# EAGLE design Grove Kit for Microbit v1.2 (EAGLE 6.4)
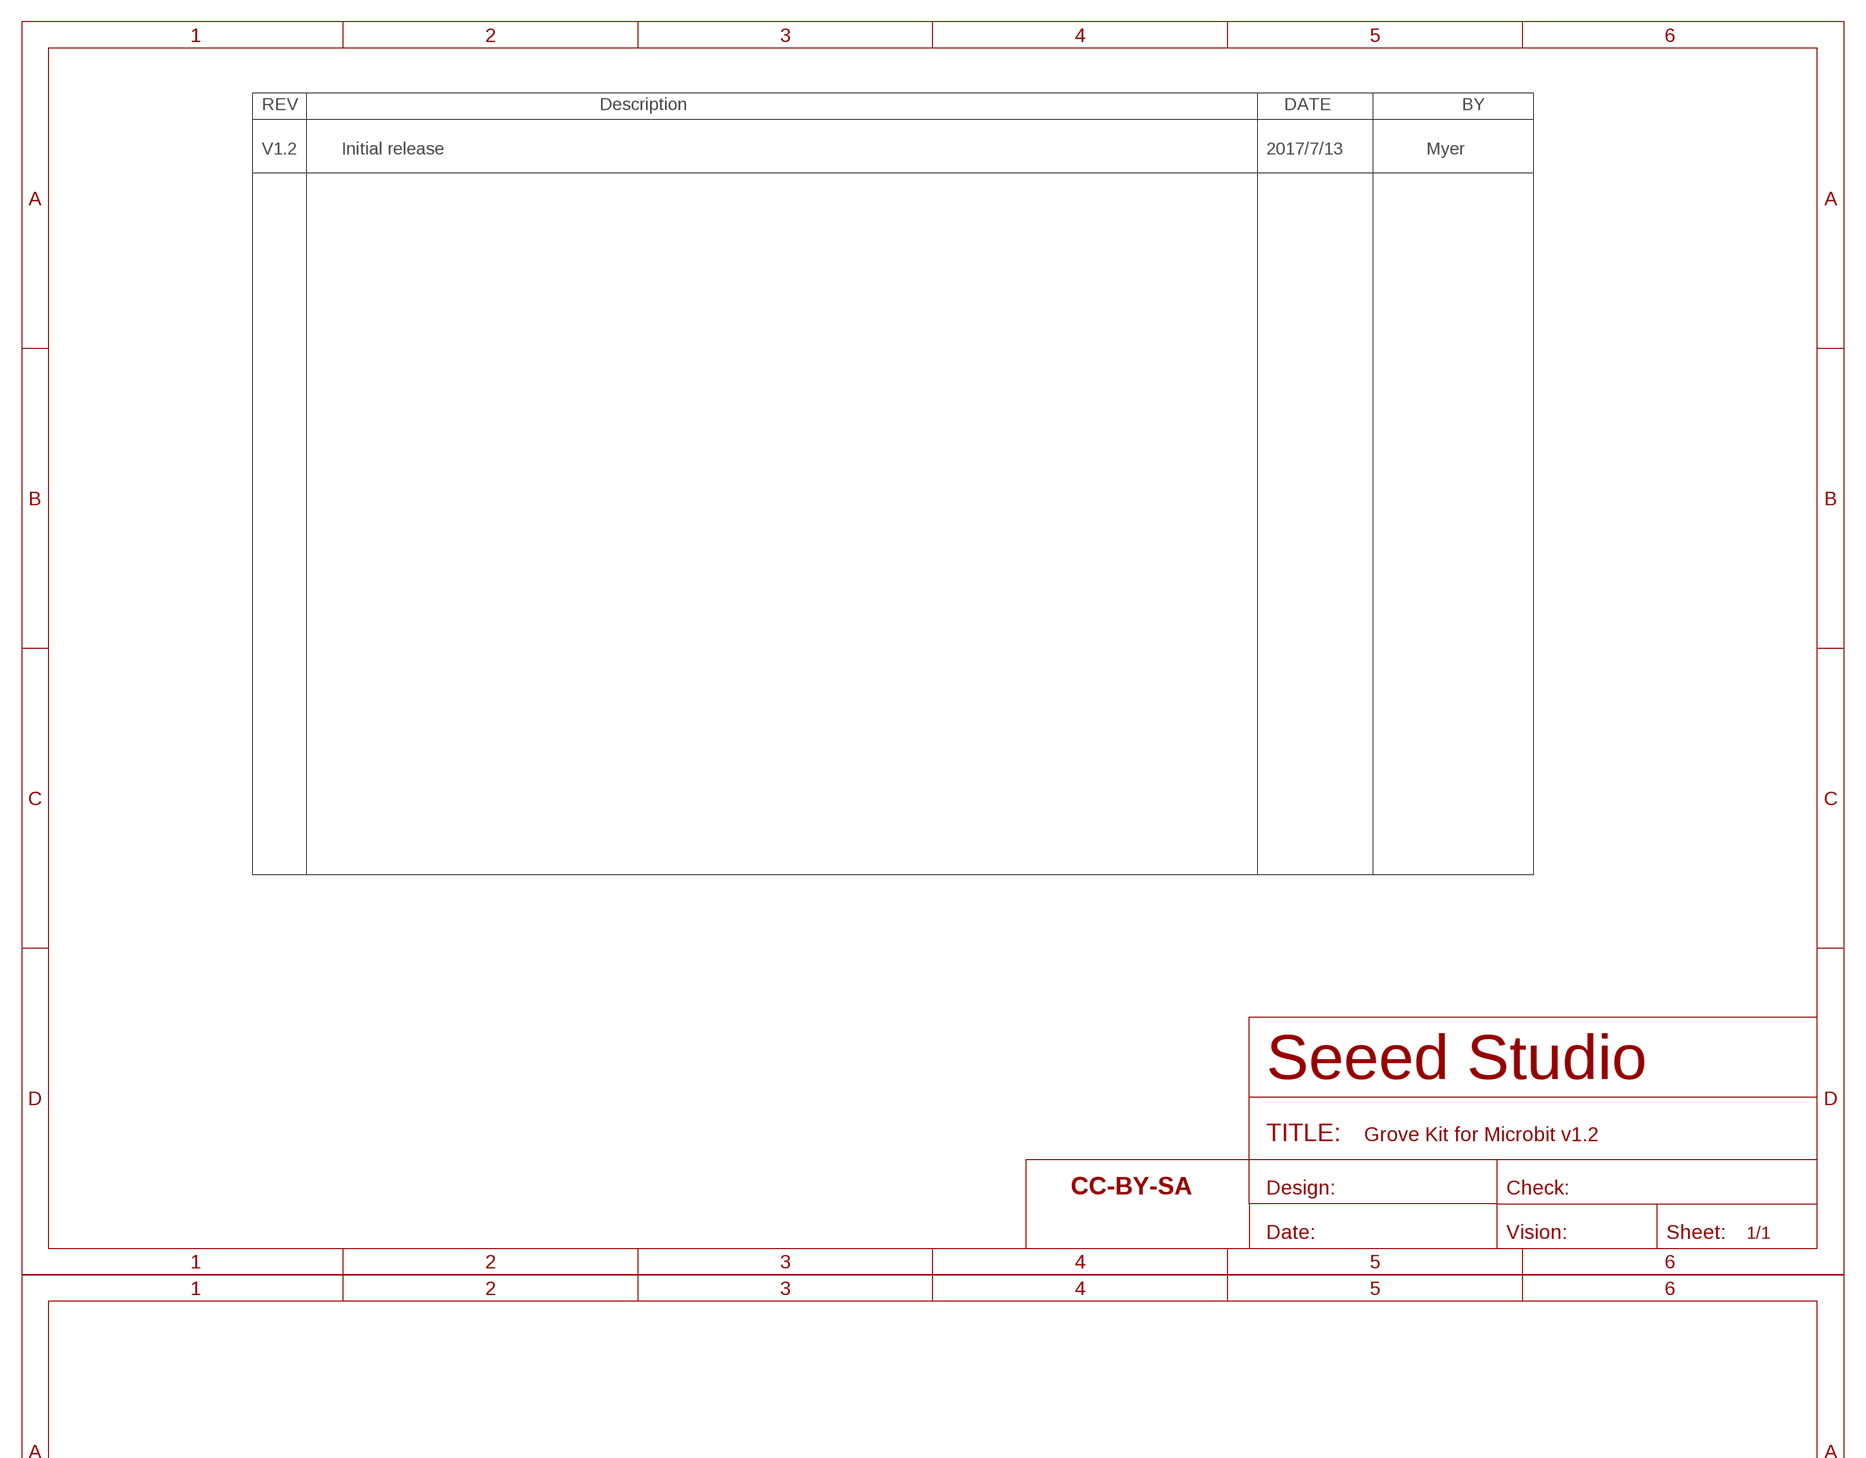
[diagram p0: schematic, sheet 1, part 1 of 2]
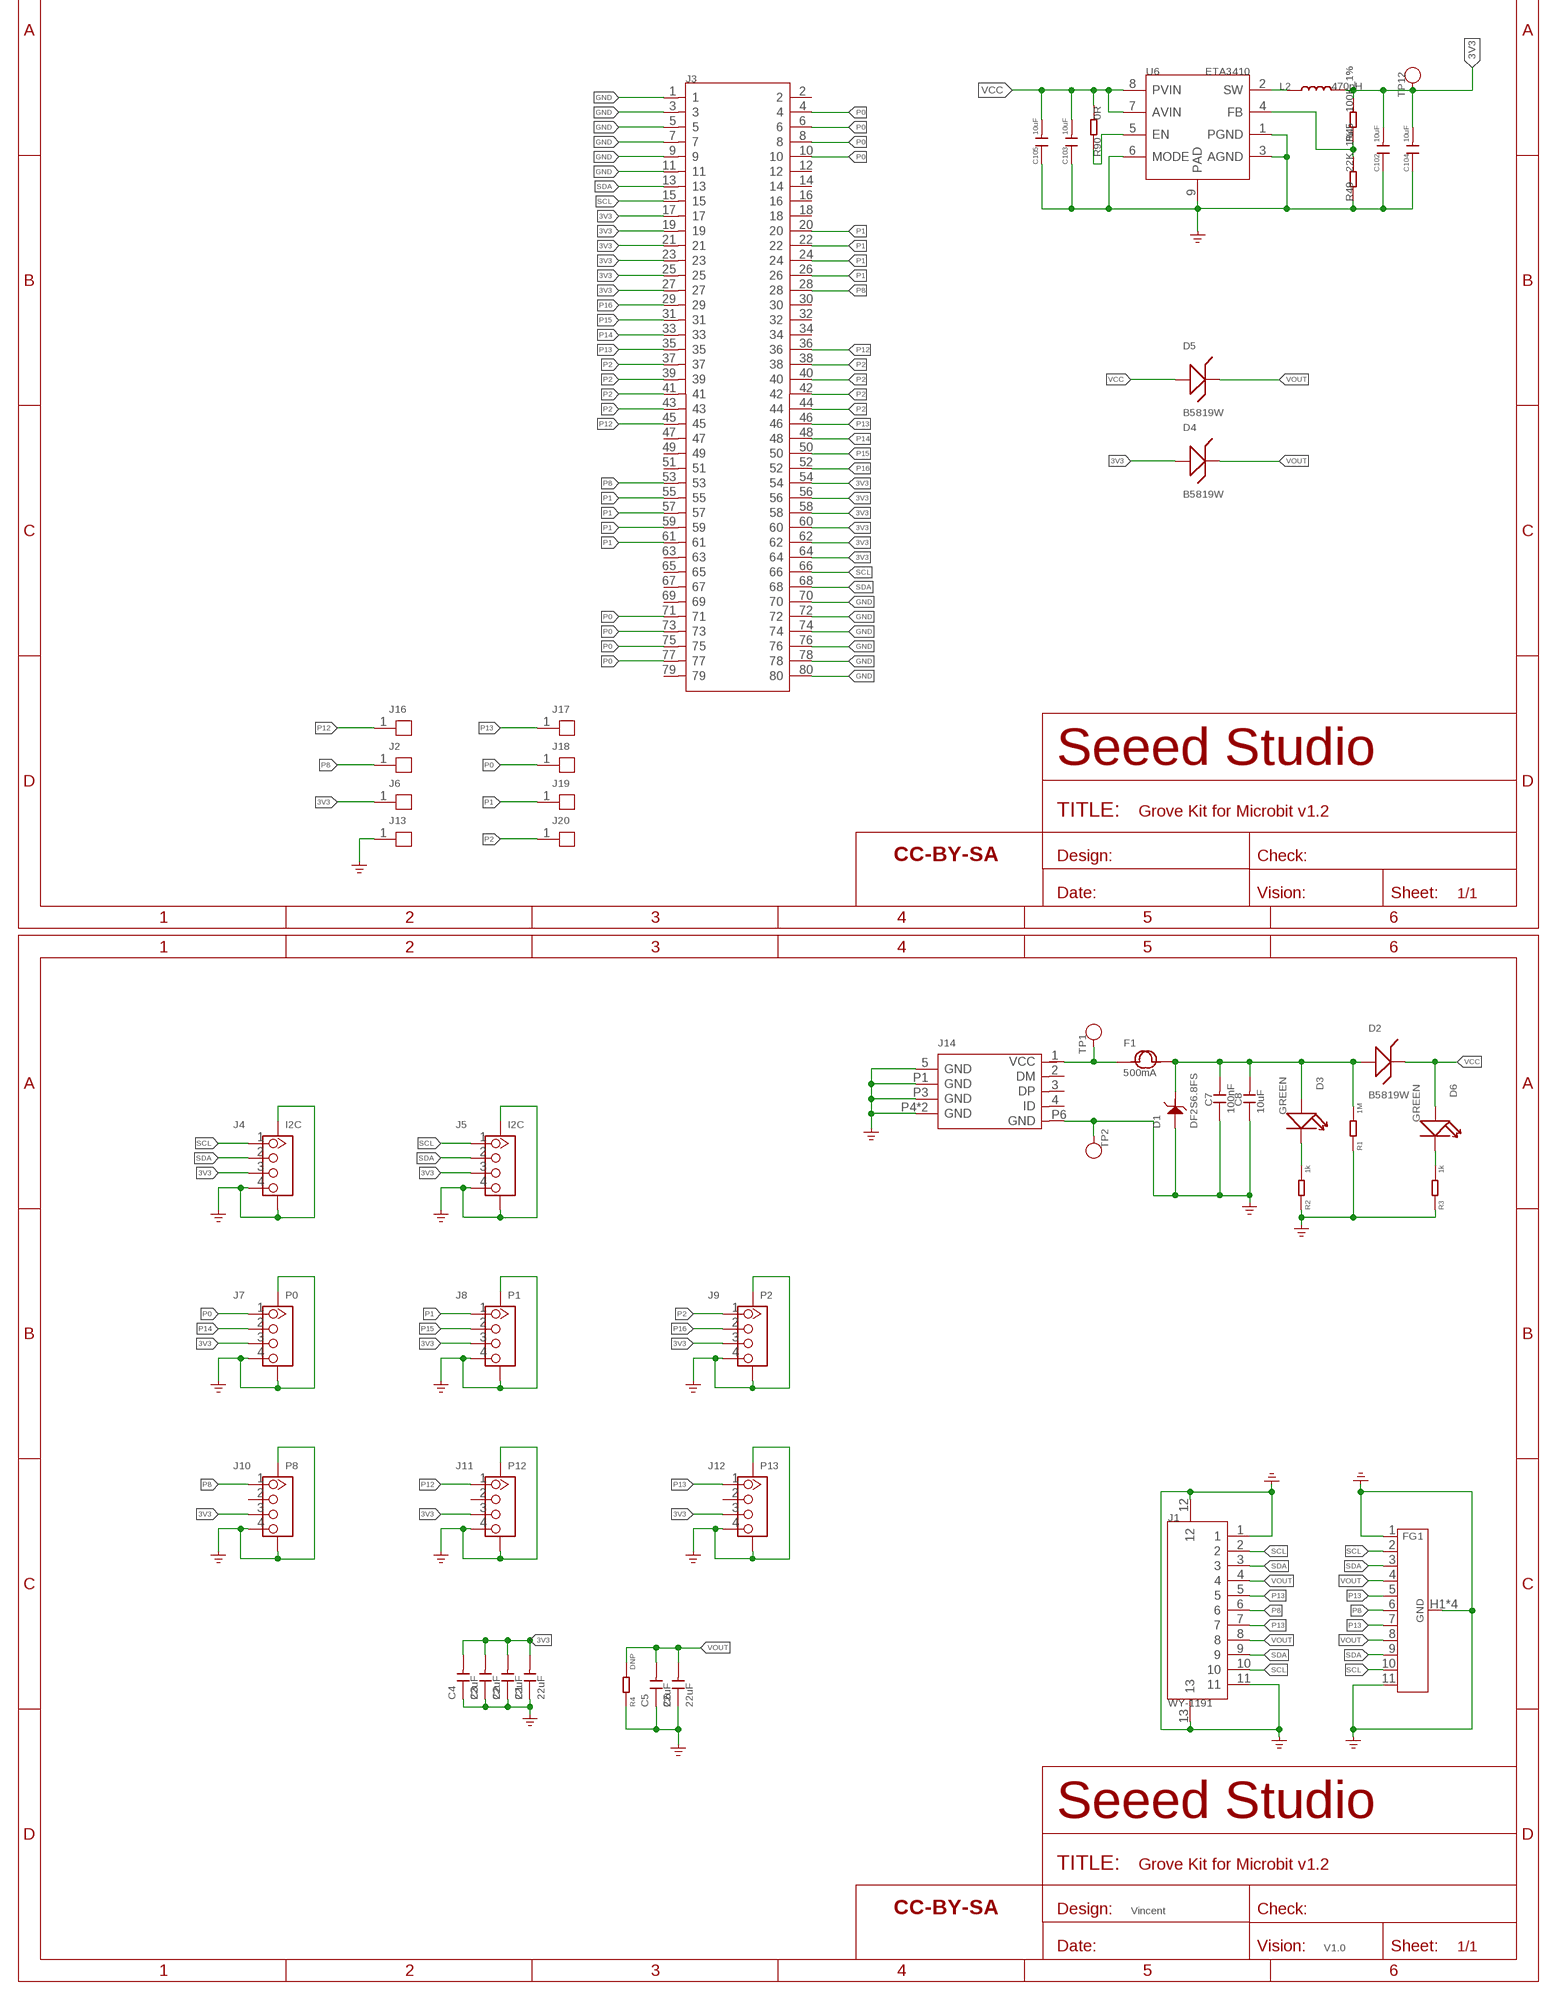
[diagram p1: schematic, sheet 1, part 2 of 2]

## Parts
C1  22uF  CAP-0805  [C0805]
C2  22uF  CAP-0805  [C0805]
C3  22uF  CAP-0805  [C0805]
C4  22uF  CAP-0805  [C0805]
C5  22uF  CAP-0805  [C0805]
C6  22uF  CAP-0805  [C0805]
C7  100nF  C-0402  [C0402]
C8  10uF  C-0603  [C0603]
C102  10uF  C-0603  [C0603]
C103  10uF  C-0603  [C0603]
C104  10uF  C-0603  [C0603]
C105  10uF  C-0603  [C0603]
D1  DF2S6.8FS  D-ESD-2P'DF2S6.8FS'  [SOD-923]
D2  B5819W  D-ZENER-2P'MMSZ4689-V'  [SOD-123]
D3  GREEN  LED-0402  [LED-0402]
D4  B5819W  D-ZENER-2P'MMSZ4689-V'  [SOD-123]
D5  B5819W  D-ZENER-2P'MMSZ4689-V'  [SOD-123]
D6  GREEN  LED-0402  [LED-0402]
F1  500mA  FUSE'1206'  [F1206]
FG1  HALF_FINGER  [HALF_FINGER]
FR1  SEEEDSTUDIO-OPEN-SCH-FRAME  [SEEEDSTUDIO-PCB-FRAME]
FR2  SEEEDSTUDIO-OPEN-SCH-FRAME  [SEEEDSTUDIO-PCB-FRAME]
FR3  SEEEDSTUDIO-OPEN-SCH-FRAME  [SEEEDSTUDIO-PCB-FRAME]
J1  WY-1191  HEADER-11P-SMD  [H11P-SMD-1.0-13.5X4.35X3.1MM]
J2  HEADER-1P-3.9MM  [1P-DIP-8X5MM]
J3  CONNECTOR-MICRO-BIT-2X40P  [CONNECTOR2X40P-1.27-57X14]
J4  I2C  GROVE-CONNECTOR-SMD'90D'  [HW4-SMD-2.0-90D]
J5  I2C  GROVE-CONNECTOR-SMD'90D'  [HW4-SMD-2.0-90D]
J6  HEADER-1P-3.9MM  [1P-DIP-8X5MM]
J7  P0  GROVE-CONNECTOR-SMD'90D'  [HW4-SMD-2.0-90D]
J8  P1  GROVE-CONNECTOR-SMD'90D'  [HW4-SMD-2.0-90D]
J9  P2  GROVE-CONNECTOR-SMD'90D'  [HW4-SMD-2.0-90D]
J10  P8  GROVE-CONNECTOR-SMD'90D'  [HW4-SMD-2.0-90D]
J11  P12  GROVE-CONNECTOR-SMD'90D'  [HW4-SMD-2.0-90D]
J12  P13  GROVE-CONNECTOR-SMD'90D'  [HW4-SMD-2.0-90D]
J13  HEADER-1P-3.9MM  [1P-DIP-8X5MM]
J14  MICRO-USB5+4P  [MICRO-USB5+5P-SMD-0.65-7.2X5.06MM]
J16  HEADER-1P-3.9MM  [1P-DIP-8X5MM]
J17  HEADER-1P-3.9MM  [1P-DIP-8X5MM]
J18  HEADER-1P-3.9MM  [1P-DIP-8X5MM]
J19  HEADER-1P-3.9MM  [1P-DIP-8X5MM]
J20  HEADER-1P-3.9MM  [1P-DIP-8X5MM]
L2  470nH  L-MPM201610SR33_T  [L201610]
R1  1M  R-0402  [R0402]
R2  1k  R-0402  [R0402]
R3  1k  R-0402  [R0402]
R4  DNP  R-0402  [R0402]
R45  100K_1%  R-0402  [R0402]
R49  22K_1%  R-0402  [R0402]
R90  0R  R-0402  [R0402]
TP1  TEST-POINT'4545'  [TP-D45MIL]
TP2  TEST-POINT'4545'  [TP-D45MIL]
TP12  TEST-POINT'4545'  [TP-D45MIL]
U6  ETA3410  CONVERTER-ETA3410  [DFN8G-0.5-2X2MM]

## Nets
3V3: C1.2 C2.2 C3.2 C4.2 C102.2 C104.2 D4.+ J3.17 J3.19 J3.21 J3.23 J3.25 J3.27 J3.54 J3.56 J3.58 J3.60 J3.62 J3.64 J4.3 J5.3 J6.1 J7.3 J8.3 J9.3 J10.3 J11.3 J12.3 L2.2 R45.2 TP12.T
GND: C1.1 C2.1 C3.1 C4.1 C5.1 C6.1 C7.1 C8.1 C102.1 C103.1 C104.1 C105.1 D1.2 FG1.1 FG1.11 FG1.H1 FG1.H2 FG1.P2 FG1.P4 J1.1 J1.11 J1.12 J1.13 J3.1 J3.3 J3.5 J3.7 J3.9 J3.11 J3.70 J3.72 J3.74 J3.76 J3.78 J3.80 J4.4 J4.SS1 J4.SS2 J5.4 J5.SS1 J5.SS2 J7.4 J7.SS1 J7.SS2 J8.4 J8.SS1 J8.SS2 J9.4 J9.SS1 J9.SS2 J10.4 J10.SS1 J10.SS2 J11.4 J11.SS1 J11.SS2 J12.4 J12.SS1 J12.SS2 J13.1 J14.5(GND) J14.P1(GND) J14.P3(GND) J14.P4(GND) J14.P5(GND) J14.P6(GND) R1.1 R2.1 R3.1 R4.1 R49.1 TP2.T U6.1(PGND) U6.3(AGND) U6.6(MODE) U6.9(PAD) ; supply symbol labelled GND_POWER
N$1: D6.- R3.2
N$2: D3.- R2.2
N$3: C7.2 C8.2 D1.1 D2.+ D3.+ F1.2 R1.2
N$17: R90.1 U6.5(EN)
N$24: F1.1 J14.1(VCC) TP1.T
N$48: L2.1 U6.2(SW)
N$49: R45.1 R49.2 U6.4(FB)
P0: J3.4 J3.6 J3.8 J3.10 J3.71 J3.73 J3.75 J3.77 J7.1 J18.1
P1: J3.20 J3.22 J3.24 J3.26 J3.55 J3.57 J3.59 J3.61 J8.1 J19.1
P2: J3.37 J3.38 J3.39 J3.40 J3.41 J3.42 J3.43 J3.44 J9.1 J20.1
P8: FG1.6 J1.6 J2.1 J3.28 J3.53 J10.1
P12: J3.36 J3.45 J11.1 J16.1
P13: FG1.5 FG1.7 J1.5 J1.7 J3.35 J3.46 J12.1 J17.1
P14: J3.33 J3.48 J7.2
P15: J3.31 J3.50 J8.2
P16: J3.29 J3.52 J9.2
SCL: FG1.2 FG1.10 J1.2 J1.10 J3.15 J3.66 J4.1 J5.1
SDA: FG1.3 FG1.9 J1.3 J1.9 J3.13 J3.68 J4.2 J5.2
VCC: C103.2 C105.2 D2.- D5.+ D6.+ R90.2 U6.7(AVIN) U6.8(PVIN)
VOUT: C5.2 C6.2 D4.- D5.- FG1.4 FG1.8 J1.4 J1.8 R4.2
Unconnected: J3.2 J3.12 J3.14 J3.16 J3.18 J3.30 J3.32 J3.34 J3.47 J3.49 J3.51 J3.63 J3.65 J3.67 J3.69 J3.79 J10.2 J11.2 J12.2 J14.2(DM) J14.3(DP) J14.4(ID)

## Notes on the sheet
- V1.2 | Initial release | 2017/7/13 | Myer
- Vincent
- V1.0

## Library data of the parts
C1-C6 = Discrete-new:CAP: Ceramic Capacitors
C7 C8 C102-C105 = Discrete-small:C*: Ceramic Capacitors
D1 = Discrete-new:D-ESD-2P: SOD-923:304060009;SOD-123:304060001
D2 D4 D5 = Discrete-new:D-ZENER-2P: SOD-123:304030008;SOT-23:304030000
D3 D6 = Discrete-new:LED
F1 = Discrete-new:FUSE
FG1 = G2-Xadow3:HALF_FINGER
FR1-FR3 = moudle-new:SEEEDSTUDIO-OPEN-SCH-FRAME
J1 = Connector-new:HEADER-11P-SMD
J2 J6 J13 J16-J20 = Connector-new:HEADER-1P
J3 = Connector-new:CONNECTOR-MICRO-BIT-2X40P
J4 J5 J7-J12 = Connector-new:GROVE-CONNECTOR-SMD: 4P-SMD-2.0:320110030;4P-SMD-2.0-90D:320110032
J14 = Connector-new:MICRO-USB5+4P: 5+4P-SMD-0.65-B:320010000;5+2P-SMD-0.65-AB:340032001;5+5P-SMD-0.65-7.2X5.06MM:320010050;
L2 = Discrete-new:L
R1-R4 R45 R49 R90 = Discrete-small:R*
TP1 TP2 TP12 = Discrete-new:TEST-POINT; PARTNO: DNP
U6 = IC-new:CONVERTER-ETA3410: 3MHZ 2A High Step-Down Converter in DFN2x2-8L Package

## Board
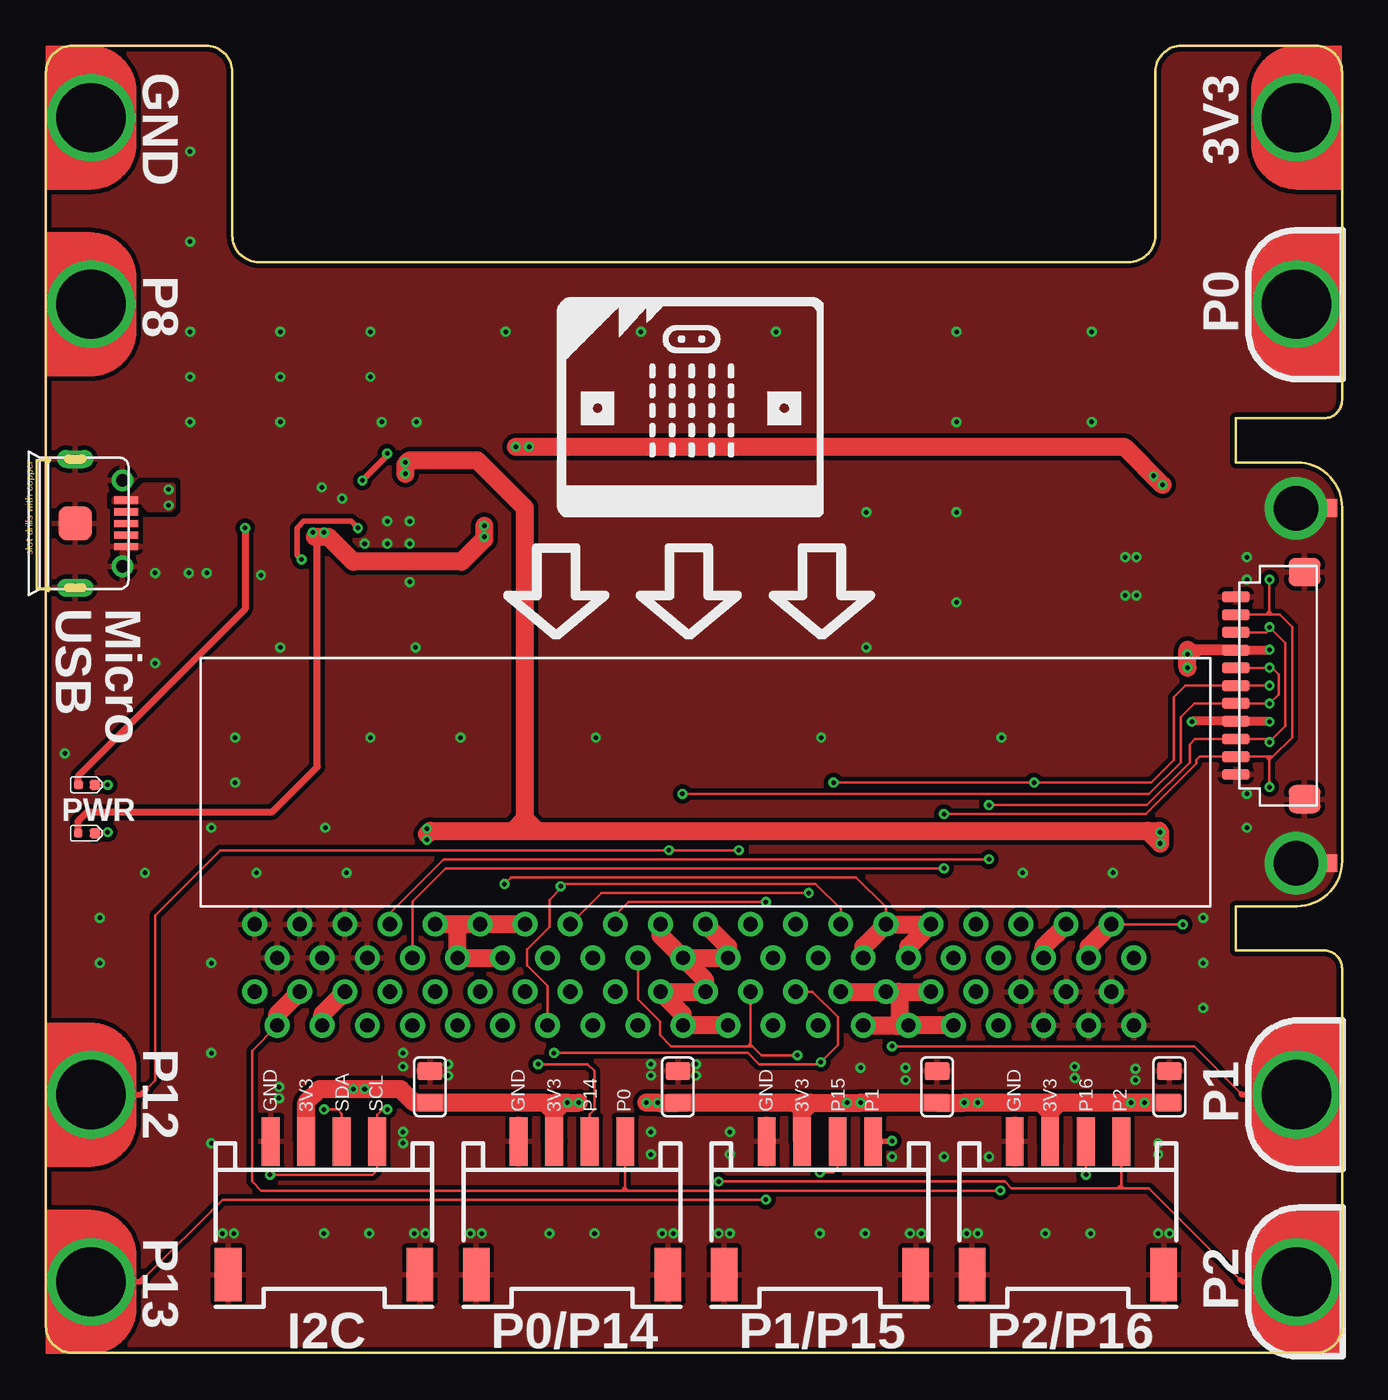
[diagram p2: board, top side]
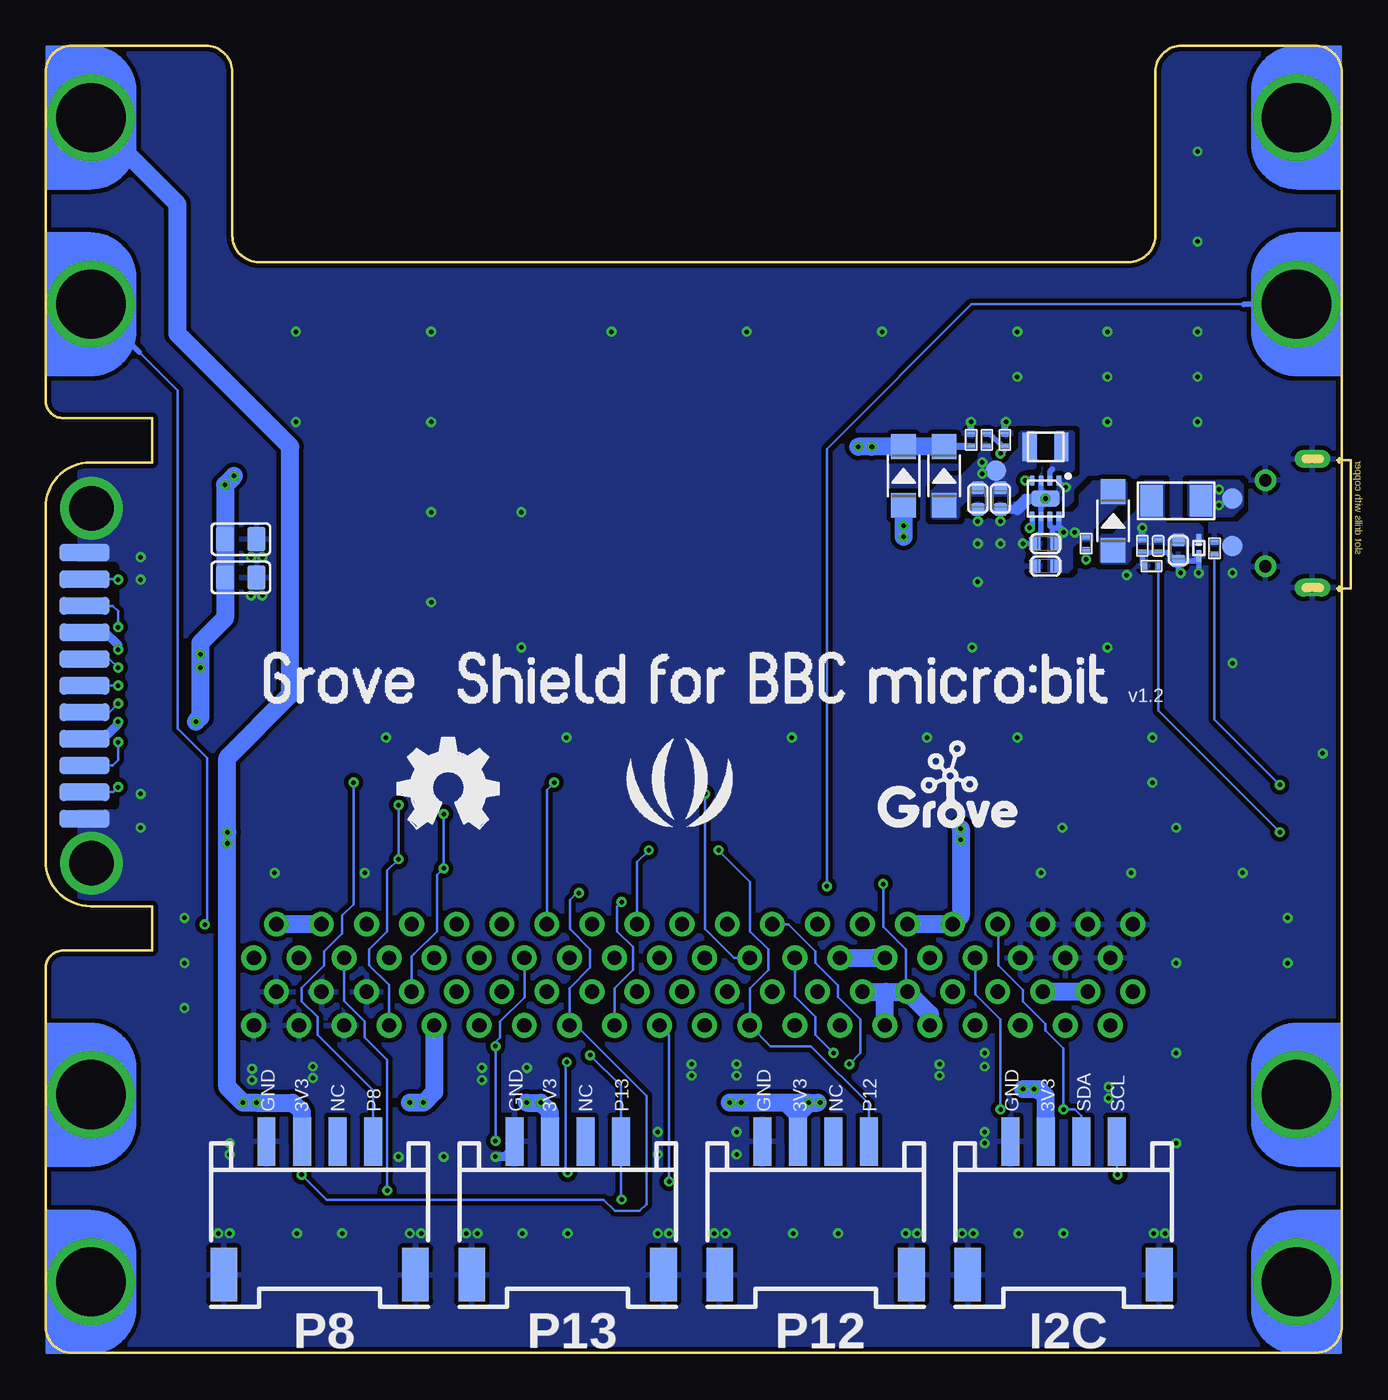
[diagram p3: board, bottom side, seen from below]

Size 73.03 x 73.65 mm. Coordinates in mm from the lower left corner, seen from the top.
Outline: 71.53,0 arc90 73.03,1.49 73.03,21.67 arc90 72.03,22.67 67.03,22.67 67.03,25.17 70.49,25.17 arc90 73.03,27.71 73.03,47.63 arc90 70.49,50.17 67.03,50.17 67.03,52.67 72.03,52.67 arc90 73.03,53.67 73.03,72.16 arc90 71.53,73.65 64,73.65 arc90 62.5,72.15 62.5,62.95 arc-90 61,61.45 12,61.45 arc-90 10.5,62.95 10.5,72.15 arc90 9,73.65 1.5,73.65 arc90 0,72.15
Outline: 0,72.14 0,1.5 arc90 1.5,0 71.54,0
Copper layers (1*16): Top 0.035mm / dielectric 1.5mm / Bottom 0.035mm
Design rules "SeeedStudio_2layer_DRU_no_angle_20140221 *": minimum track width 1mil, minimum drill 10mil, track to track 5mil, track to pad 5mil, pad to pad 5mil, via to via 5mil, smd to smd 0mil, copper to edge 10mil, drill to drill 10mil, minimum pad ring 10mil, minimum via ring 6mil, stop-mask expansion 2mil, vias tented up to drill 25mil, thermal gap 10mil
bRestrict: area 16.4,50.5 to 16.9,51.9

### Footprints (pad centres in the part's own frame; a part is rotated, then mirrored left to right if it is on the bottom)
C0805 = smd 1.397 x 1.016: 1 0,0.889; 2 0,-0.889
C0402 = smd 0.508 x 0.385: 1 0,0.383; 2 0,-0.383
C0603 = smd 0.762 x 0.696: 1 0,0.602; 2 0,-0.602
SOD-923 = smd 0.7 x 0.3: 1 -0.45,0; 2 0.45,0
SOD-123 = smd 1.397 x 1.397: + -1.651,0; - 1.651,0
LED-0402 = smd 0.5 x 0.5: + -0.463,0 | smd 0.58 x 0.58: - 0.468,0
F1206 = smd 1.27 x 1.778: 1 -1.397,0; 2 1.397,0
HALF_FINGER = smd 2.8 x 1 bottom: 1 3.8,7.5; 2 3.8,6; 3 3.8,4.5; 4 3.8,3; 5 3.8,1.5; 6 3.8,0; 7 3.8,-1.5; 8 3.8,-3; 9 3.8,-4.5; 10 3.8,-6; 11 3.8,-7.5 | drill 2.5 pad 3.516: H1 3.4,10; H2 3.4,-10 | smd 1.27 x 1: P2 5.1,10; P4 5.1,-10
H11P-SMD-1.0-13.5X4.35X3.1MM = smd 0.6 x 1.55: 1 -5,0; 2 -4,0; 3 -3,0; 4 -2,0; 5 -1,0; 6 0,0; 7 1,0; 8 2,0; 9 3,0; 10 4,0; 11 5,0 | smd 1.6 x 1.8: 12 -6.4,3.875; 13 6.4,3.875
1P-DIP-8X5MM = drill 3.9: 1 0,0
CONNECTOR2X40P-1.27-57X14 = drill 0.8 pad 1.4: 1 24.13,0; 2 24.13,3.8; 3 22.86,1.9; 4 22.86,5.7; 5 21.59,0; 6 21.59,3.8; 7 20.32,1.9; 8 20.32,5.7; 9 19.05,0; 10 19.05,3.8; 11 17.78,1.9; 12 17.78,5.7; 13 16.51,0; 14 16.51,3.8; 15 15.24,1.9; 16 15.24,5.7; 17 13.97,0; 18 13.97,3.8; 19 12.7,1.9; 20 12.7,5.7; 21 11.43,0; 22 11.43,3.8; 23 10.16,1.9; 24 10.16,5.7; 25 8.89,0; 26 8.89,3.8; 27 7.62,1.9; 28 7.62,5.7; 29 6.35,0; 30 6.35,3.8; 31 5.08,1.9; 32 5.08,5.7; 33 3.81,0; 34 3.81,3.8; 35 2.54,1.9; 36 2.54,5.7; 37 1.27,0; 38 1.27,3.8; 39 0,1.9; 40 0,5.7; 41 -1.27,0; 42 -1.27,3.8; 43 -2.54,1.9; 44 -2.54,5.7; 45 -3.81,0; 46 -3.81,3.8; 47 -5.08,1.9; 48 -5.08,5.7; 49 -6.35,0; 50 -6.35,3.8; 51 -7.62,1.9; 52 -7.62,5.7; 53 -8.89,0; 54 -8.89,3.8; 55 -10.16,1.9; 56 -10.16,5.7; 57 -11.43,0; 58 -11.43,3.8; 59 -12.7,1.9; 60 -12.7,5.7; 61 -13.97,0; 62 -13.97,3.8; 63 -15.24,1.9; 64 -15.24,5.7; 65 -16.51,0; 66 -16.51,3.8; 67 -17.78,1.9; 68 -17.78,5.7; 69 -19.05,0; 70 -19.05,3.8; 71 -20.32,1.9; 72 -20.32,5.7; 73 -21.59,0; 74 -21.59,3.8; 75 -22.86,1.9; 76 -22.86,5.7; 77 -24.13,0; 78 -24.13,3.8; 79 -25.4,1.9; 80 -25.4,5.7
HW4-SMD-2.0-90D = smd 1.01 x 2.74: 1 -3,-0.1; 2 -1,-0.1; 3 1,-0.1; 4 3,-0.1 | smd 1.5 x 3: SS1 -5.4,7.4; SS2 5.4,7.4
MICRO-USB5+5P-SMD-0.65-7.2X5.06MM = smd 0.4 x 1.35: 1 -1.3,2.875; 2 -0.65,2.875; 3 0,2.875; 4 0.65,2.875; 5 1.3,2.875 | smd 1.9 x 1.9: P1 0,0 | drill 0.508 pad 1.016 long: P3 -3.625,0; P4 3.625,0 | drill 0.7: P5 -2.425,2.65; P6 2.425,2.65
L201610 = smd 0.8 x 1.6: 1 -0.9,0; 2 0.9,0
R0402 = smd 0.508 x 0.385: 1 0,0.383; 2 0,-0.383
TP-D45MIL = smd 1.143 x 1.143: T 0,0
DFN8G-0.5-2X2MM = smd 0.6 x 0.3: 1 -1,0.75; 2 -1,0.25; 3 -1,-0.25; 4 -1,-0.75; 5 1,-0.75; 6 1,-0.25; 7 1,0.25; 8 1,0.75 | smd 0.9 x 1.6: 9 0,0

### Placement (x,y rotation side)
C1  35.61,14.99 0 top
C2  50.21,14.99 0 top
C3  21.64,14.99 0 top
C4  63.3,14.99 0 top
C5  62.03,43.69 270 bottom
C6  62.03,45.85 270 bottom
C7  10.34,45.47 180 bottom
C8  9.19,45.21 180 bottom
C102  20.5,48.13 180 bottom
C103  16.69,44.32 90 bottom
C104  19.23,48.13 180 bottom
C105  16.69,45.59 90 bottom
D1  8.05,45.34 270 bottom
D2  12.88,46.87 90 bottom
D3  2.29,32 0 top
D4  22.4,49.4 90 bottom
D5  24.69,49.4 90 bottom
D6  2.28,29.27 0 top
F1  9.32,48.01 180 bottom
FG1  67.03,37.59 0 top
FR1  not placed on the board
FR2  not placed on the board
FR3  not placed on the board
J1  67.03,37.59 270 top
J2  2.54,59.08 180 top
J3  37.16,18.45 0 top
J4  15.67,11.81 180 top
J5  15.67,11.81 180 bottom
J6  70.46,69.6 0 top
J7  29.64,11.81 180 top
J8  43.61,11.81 180 top
J9  57.58,11.81 180 top
J10  57.58,11.81 180 bottom
J11  29.64,11.81 180 bottom
J12  43.61,11.81 180 bottom
J13  2.54,69.6 180 top
J14  1.65,46.74 270 top
J16  2.54,14.55 180 top
J17  2.54,4 180 top
J18  70.46,59.08 0 top
J19  70.46,14.55 0 top
J20  70.46,4 0 top
L2  16.69,51.05 180 bottom
R1  11.24,45.47 180 bottom
R2  7.16,45.34 0 bottom
R3  10.72,44.33 90 bottom
R4  20.88,51.44 0 bottom
R45  19.99,51.44 0 bottom
R49  18.97,51.44 0 bottom
R90  14.4,45.59 180 bottom
TP1  6.16,48.13 180 bottom
TP2  6.16,45.47 180 bottom
TP12  19.48,49.72 180 bottom
U6  16.69,48.13 270 bottom
U$13  [OSHW_FILLX200_NOTEXT_TNAME]  53.18,29.56 0 bottom
U$14  [SEEED-SILK-TNAME-280*268MIL]  37.3,31.34 0 bottom

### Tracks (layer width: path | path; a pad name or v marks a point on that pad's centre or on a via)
3V3  (via drill 0.25 pad 0.51)
  Top 0.305: v21.46,28.9 21.46,29.21 | v21.46,29.54 21.46,29.26 21.49,29.24
  Top 1.016: 26.97,29.41 21.66,29.41 21.49,29.24 21.46,29.21 | 26.97,29.41 62.08,29.41 | 62.08,29.41 62.71,29.41 v62.79,29.34 v62.79,28.7 62.08,29.41 | J3.58 J3.62 23.19,24.12 23.16,24.15 | J3.56 J3.60 23.16,24.15 | J3.17 48.22,18.45 48.16,18.52 | 48.16,18.52 48.13,18.54 48.13,20.28 48.05,20.35 | 48.05,20.35 J3.23 J3.27 | 48.05,20.35 J3.19 | J3.25 47.93,18.45 | 48.02,18.45 J3.21 47.93,18.45 | 48.16,18.52 48.05,18.41 47.96,18.41 47.93,18.45 | 42.21,14.1 42.59,14.1 | 42.59,14.1 43.1,14.1 | J8.3 42.61,14.08 42.59,14.1 | 42.21,14.1 42.59,13.72 | 43.1,14.1 42.59,13.59 | v33.83,14.1 v34.47,14.1 C1.2 42.21,14.1 | 28.12,14.1 28.75,14.1 | 28.75,14.1 v29.39,14.1 | v29.39,14.1 v30.02,14.1 | J7.3 28.64,13.99 28.75,14.1 | 28.12,14.1 28.62,13.59 29.13,14.1 v29.39,14.1 | J4.3 14.67,14.11 15.42,14.86 v17.32,14.86 19.99,14.86 20.75,14.1 C3.2 28.12,14.1 | v61.14,14.1 56.69,14.1 | 56.69,14.1 56.06,14.1 | 56.06,14.1 v52.5,14.1 v51.74,14.1 C2.2 v45.9,14.1 43.1,14.1 | J9.3 56.58,13.99 56.69,14.1 | 56.06,14.1 56.44,13.72 | v61.14,14.1 57.07,14.1 56.69,13.72 | C4.2 v61.14,14.1 | 26.97,30.1 26.97,47.62 24.31,50.29 20.5,50.29 20.24,50.04 v20.24,49.53 | 26.97,30.1 26.97,29.41 | 26.97,30.1 26.34,29.46 | 26.97,30.1 27.61,29.46 | 23.16,24.15 J3.64 21.89,24.13
  Bottom 0.508: 29.51,14.1 v29.39,14.1
  Bottom 1.016: v52.5,14.1 v51.74,14.1 51.13,14.71 J3.17 | J3.60 J3.64 21.46,24.61 v21.46,29.54 | J3.54 26.34,22.25 | 26.34,22.25 J3.58 | J12.3 44.61,13.57 v45.13,14.1 v45.9,14.1 | J11.3 30.64,13.48 v30.02,14.1 | v30.02,14.1 29.51,14.1 | v30.02,14.1 31.29,14.1 | 31.29,14.1 v34.47,14.1 | 31.29,14.1 30.66,13.46 | J10.3 58.58,13.57 59.1,14.1 v61.14,14.1 v61.9,14.1 62.79,14.99 v62.79,29.34 62.79,33.53 59.23,37.08 59.23,51.05 65.58,57.4 65.58,64.71 J6.1 | J5.3 16.67,14.46 17.07,14.86 v17.32,14.86 v17.96,14.86 | 26.35,22.26 26.34,22.25
  other vias: 20.24,50.17
  pour Bottom (isolate 0.254, no thermals): 23.04,46.99 21.64,46.99 21.51,47.12 21.51,47.62 20.88,48.26 18.46,48.26 18.21,48.51 18.21,49.33 17.75,49.78 17.32,49.78 17.19,49.91 17.19,51.82 17.32,51.94 18.08,51.94 18.21,51.82 18.21,50.98 18.89,50.29 19.3,50.29 19.41,50.29 19.61,50.48 19.61,51.13 19.79,51.31 20.21,51.31 20.5,51.02 20.5,50.37 21.46,49.4 22.27,49.4 23.16,48.51 23.16,47.12
GND  (via drill 0.25 pad 0.51)
  Bottom 0.305: 17.29,45.88 17.32,45.85 | 17.29,45.88 C105.1 v17.96,45.59 | 17.29,45.88 16.94,46.23 U6.6 16.94,47.88 U6.9 16.94,48.38 U6.3 | U6.1 15.94,49.03 15.67,48.77 v15.54,48.77 | R3.1 11.24,44.47 R1.1 C7.1 9.83,45.08 9.35,44.61 C8.1 | D1.2 8.05,44.83 | 8.05,44.83 v8.05,43.94 | C8.1 8.27,44.61 8.05,44.83 | C8.1 9.19,44.07 v9.07,43.94
  Bottom 0.406: R4.1 v20.88,52.45 | R49.1 18.97,52.39 v18.91,52.45
  Bottom 0.508: C104.1 18.43,47.53 17.83,48.13 17.57,48.13 | 17.57,48.13 U6.9 | 17.57,48.13 18.27,47.43 | J12.4 46.61,11.61 47.17,11.05 v47.67,11.05
  other vias: 19.23,46.86 20.5,46.86 19.23,45.59 20.5,45.59 20.5,43.43 16.69,48.13 20.11,16.89 20.11,16.13 22.65,15.62 22.65,16.26 61.39,16 61.39,15.37 34.09,15.62 34.09,16.26 36.62,16.26 36.62,15.62 57.96,15.49 57.96,16.13 48.44,15.37 48.44,16.07 38.53,12.45 38.53,11.18 50.6,11.05 53.14,11.05 20.11,12.45 20.11,11.81 13.13,14.99 13.13,14.35 9.96,6.73 10.59,6.73 20.75,6.73 21.38,6.73 23.93,6.73 24.56,6.73 34.09,12.45 34.09,11.18 34.72,6.73 35.36,6.73 37.9,6.73 38.53,6.73 48.69,6.73 49.33,6.73 51.87,6.73 52.5,6.73 62.66,6.73 63.3,6.73 62.66,11.81 62.66,11.18 67.67,31.5 67.67,29.59 67.67,43.56 67.67,44.83 45.9,16.07 9.32,16.89 9.32,11.81 9.32,29.59 8.12,62.61 8.12,67.69 55.04,27.05 60.12,27.05 65.2,24.51 65.2,21.97 65.2,19.43 9.32,21.97 61.45,42.67 60.81,42.67 60.81,44.83 61.45,44.83 6.15,43.94 12.11,43.82 8.12,57.53 13.2,57.53 18.28,57.53 18.28,54.99 13.2,54.99 8.12,54.99 8.12,52.45 13.2,52.45 25.9,57.53 33.52,57.53 41.14,57.53 51.3,57.53 58.92,57.53 58.92,52.45 51.3,52.45 51.3,47.37 51.3,42.29 15.74,29.59 18.28,34.67 23.36,34.67 30.98,34.67 43.68,34.67 53.84,34.67 3.04,24.51 5.58,27.05 3.04,21.97 10.66,32.13 10.66,34.67 13.2,39.75 20.82,39.75 46.22,47.37 46.22,39.75 6.15,38.86 1.06,33.78 15.67,6.73 28.37,6.73 30.91,6.73 43.61,6.73 46.15,6.73 56.31,6.73 58.85,6.73 18.21,6.73 11.86,27.05 16.94,27.05
  pour Top (isolate 0.254, rank 6): -0.21,74.04 73.45,74.04 73.45,-0.25 -0.21,-0.25
  pour Bottom (isolate 0.254, rank 6): -0.21,74.04 73.45,74.04 73.45,-0.25 -0.21,-0.25
N$1  (via drill 0.25 pad 0.51)
  Top 0.127: D6.- 3.41,29.27 v3.48,29.34
  Bottom 0.127: R3.2 10.33,36.19 v3.48,29.34
N$2  (via drill 0.25 pad 0.51)
  Top 0.127: v3.48,32 D3.-
  Bottom 0.127: R2.2 7.16,35.69 v3.48,32
N$3  (via drill 0.25 pad 0.51)
  Top 0.406: v11.22,46.48 11.22,41.91 1.95,32.64 1.83,32.51 1.82,32.51 D3.+
  Bottom 0.406: R1.2 v11.24,46.47 v11.22,46.48
  pour Bottom (isolate 0.254, no thermals): 10.08,49.15 11.1,49.15 11.48,48.77 11.48,47.55 12.93,46.1 13.51,46.1 13.64,45.97 13.64,44.58 13.51,44.45 12.11,44.45 11.86,44.7 11.86,45.34 11.73,45.47 7.92,45.47 7.8,45.59 7.8,46.48 8.05,46.74 9.83,46.74 9.96,46.86 9.96,49.02
N$17  (via drill 0.25 pad 0.51)
  Top 0.305: v14.4,44.7 14.15,44.96 14.15,46.48 14.53,46.86 17.19,46.86 v17.57,46.48
  Bottom 0.305: R90.1 v14.4,44.7 | U6.5 17.44,46.62 v17.57,46.48
N$24  (via drill 0.25 pad 0.51)
  other vias: 6.91,48.64 6.91,47.75
  pour Bottom (isolate 0.254, no thermals): 8.3,47.12 6.15,47.12 5.51,47.75 5.51,48.9 5.76,49.15 8.56,49.15 8.69,49.02 8.69,47.24 8.56,47.12
  pour Top (isolate 0.254, no thermals): 3.86,48.26 4.75,48.26 5.51,49.02 7.16,49.02 7.29,48.9 7.29,47.62 7.03,47.37 5.76,47.37 5.38,47.75 3.86,47.75 3.73,47.88 3.73,48.13
N$48
  Bottom 0.305: U6.2 16.44,49.65 16.3,49.78
  pour Bottom (isolate 0.254, no thermals): 16.3,49.66 15.16,49.66 15.04,49.78 15.04,51.82 15.16,51.94 16.05,51.94 16.18,51.82 16.18,50.29 16.43,50.04 16.43,49.78
N$49  (via drill 0.25 pad 0.51)
  Top 0.305: v17.83,49.15 19.23,50.55 v19.23,50.67
  Bottom 0.305: U6.4 17.81,49.13 v17.83,49.15 | R45.1 19.86,51.82 19.1,51.05 R49.2 18.97,50.93 v19.23,50.67
P0  (via drill 0.25 pad 0.51)
  Top 0.127: v53.77,9.14 32.81,9.14 | 32.81,9.14 32.69,9.14 | 32.69,9.14 32.43,9.14 | 32.43,9.14 12.11,9.14 11.61,9.65 11.61,17.03 J3.77 | J7.1 32.64,9.35 | 32.64,9.32 32.64,9.19 32.69,9.14 | 32.64,9.35 32.43,9.14 | 32.64,9.35 32.64,9.32 | 32.64,9.32 32.81,9.14 | J3.4 64.04,24.15 v64.06,24.13
  Top 1.016: J3.77 13.03,19.08 J3.75 | J3.73 15.57,19.08 J3.71 | J3.10 56.21,22.88 J3.8 | J3.6 58.75,22.88 J3.4
  Bottom 0.127: v53.77,9.14 53.77,16.51 55.04,17.78 55.04,18.67 56.21,19.84 J3.10 | v64.06,24.13 63.93,24.26 63.93,33.53 65.58,35.18 65.58,54.23 67.74,56.39 | J18.1 70.44,59.06 70.41,59.06 68.63,57.28
  Bottom 0.305: 68.63,57.28 67.74,56.39
  Bottom 1.016: J3.75 J3.71 | J3.8 J3.4
P1  (via drill 0.25 pad 0.51)
  Top 0.127: v25.83,26.42 26.21,26.8 45.64,26.8 47.32,25.12 J3.24 | v47.67,17.27 64.69,17.27 67.36,14.61 | J19.1 68.85,14.55
  Top 0.305: J8.1 47.65,11.91 v47.67,11.94 | 68.85,14.55 67.42,14.55 67.36,14.61
  Top 1.016: J3.26 46.05,22.88 J3.24 J3.20 48.59,22.88 J3.22
  Bottom 0.127: v25.83,26.42 25.83,24 24.56,22.73 24.56,20.45 24.49,20.39 J3.59 | J3.26 46.05,20.04 47.42,18.67 47.42,17.78 47.67,17.53 v47.67,17.27 v47.67,11.94
  Bottom 1.016: J3.61 23.19,19.08 J3.59 | J3.55 25.7,20.35 | 25.7,20.35 24.53,20.35 24.49,20.39 | J3.57 25.73,20.32 25.7,20.35
P2  (via drill 0.25 pad 0.51)
  Top 0.127: J9.1 60.58,9.48 | 60.58,9.45 60.58,9.32 60.63,9.27 | v37.9,9.65 54.02,9.65 54.41,9.27 60.37,9.27 | 60.37,9.27 60.63,9.27 | 60.63,9.27 60.76,9.27 | 60.76,9.27 62.15,9.27 67.3,4.13 | 60.58,9.48 60.37,9.27 | 60.58,9.48 60.58,9.45 | 60.58,9.45 60.76,9.27 | J20.1 69.28,4
  Top 0.305: 69.28,4 67.42,4 67.3,4.13
  Top 1.016: J3.37 J3.41 35.89,19.08 J3.43 J3.39 37.16,20.98 J3.42 | J3.42 J3.38 38.43,22.88 J3.40 | J3.44 34.62,23.52 J3.42
  Bottom 0.127: v37.9,9.65 37.9,17.92 J3.37
P8  (via drill 0.25 pad 0.51)
  Top 0.127: v68.94,37.59 J1.6 64.18,37.59 63.55,36.96 63.55,33.4 62.28,32.13 v55.68,32.13 v44.37,32.13 | J3.53 28.27,20.67 27.1,21.84 27.1,22.73 28.37,24 28.37,25.53 29,26.16 v29,26.29 29.13,26.42 43.37,26.42 44.78,25 J3.28
  Bottom 0.127: v68.94,37.59 FG1.6 | v29,26.29 29,50.93 20.85,59.08 5.23,59.08 | J10.1 54.58,14.78 57.71,17.91 57.71,18.92 58.6,19.81 58.6,20.57 57.33,21.84 57.33,22.61 56.31,23.62 56.31,24.64 55.68,25.27 v55.68,32.13 | J3.28 44.78,31.72 v44.37,32.13 | 3.99,59.08 J2.1
  Bottom 0.305: 3.99,59.08 5.23,59.08 5.48,59.08 5.51,59.06
P12  (via drill 0.25 pad 0.51)
  Top 0.127: v39.04,28.32 v35.1,28.32 9.83,28.32 6.15,24.64 6.15,15.37 5.64,14.86 5.33,14.55 | J16.1 4.2,14.55
  Top 0.305: 4.2,14.55 5.33,14.55 5.64,14.86
  Bottom 0.127: 39.05,28.31 v39.04,28.32 39.7,27.66 J3.36 | J11.1 26.64,14.02 29.89,17.27 32.17,17.27 J3.45 33.35,20.55 32.31,21.59 32.31,22.73 33.32,23.75 33.32,26.54 v35.1,28.32
P13  (via drill 0.25 pad 0.51)
  Top 0.127: 39.8,17.27 39.55,17.27 | J1.5 68.92,38.59 v68.94,38.61 69.07,38.61 69.45,38.23 69.45,37.08 v68.94,36.58 68.92,36.59 J1.7 64.71,36.59 63.93,35.81 63.93,33.27 62.15,31.5 v35.86,31.5 | v40.56,8.64 9.96,8.64 5.51,4.19 | v42.34,16.76 40.31,16.76 39.8,17.27 | 39.55,17.27 35.23,17.27 34.59,17.91 34.59,18.67 33.35,19.91 J3.46 | J3.35 39.7,17.43 | 39.7,17.43 39.7,17.37 39.8,17.27 | 39.7,17.43 39.55,17.27 | 4.27,4 J17.1
  Top 0.305: 4.27,4 5.32,4 5.51,4.19
  Bottom 0.127: v68.94,38.61 69.42,39.09 FG1.5 | v68.94,36.58 69.42,36.09 FG1.7 | v40.56,8.64 40.61,8.68 J12.1 40.61,15.03 v42.34,16.76 | J3.46 34.24,22.25 35.86,23.88 v35.86,31.5
P14  (via drill 0.25 pad 0.51)
  Top 0.127: v40.56,25.4 32.81,25.4 32.08,24.66 J3.48 | J7.2 30.64,13.45 30.91,13.72 30.91,15.88 30.53,16.26 v27.73,16.26
  Bottom 0.127: v27.73,16.26 27.1,16.89 27.1,18.8 28.37,20.07 28.37,20.7 29.64,21.97 29.64,22.61 31.16,24.13 32.06,24.13 J3.48 | J3.33 40.97,20.55 39.93,21.59 39.93,22.86 40.82,23.75 40.82,25.15 v40.56,25.4
P15  (via drill 0.25 pad 0.51)
  Top 0.127: v28.62,16.89 39.55,16.89 40.18,16.26 43.53,16.26 v43.66,16.38 44.63,17.35 44.63,18.92 43.2,20.35 J3.31 | J8.2 44.61,10.4 44.37,10.16 v43.61,10.16
  Bottom 0.127: 28.64,16.88 v28.62,16.89 29.64,17.91 29.64,18.92 30.81,20.09 J3.50 | v43.66,16.38 43.74,16.3 43.74,10.29 v43.61,10.16
P16  (via drill 0.25 pad 0.51)
  Top 0.127: v42.98,25.91 31.3,25.91 J3.52 | J9.2 58.58,10.05 v58.6,10.03
  Bottom 0.127: v42.98,25.91 43.1,25.91 43.48,25.53 43.48,23.88 42.34,22.73 42.34,21.72 43.51,20.55 J3.29 43.14,18.45 39.17,14.48 39.17,8.38 39.55,8 40.94,8 41.58,8.64 57.2,8.64 v58.6,10.03
SCL  (via drill 0.25 pad 0.51)
  Top 0.127: v12.62,10.03 18.42,10.03 18.67,10.29 J4.1 18.67,13.41 18.97,13.72 v19.23,13.72 | v50.6,27.3 22.53,27.3 20.65,25.43 J3.66 | 68.94,33.59 J1.10 65.01,33.59 64.82,33.4 64.82,33.21 61.96,30.35 v50.6,30.35 | 68.94,33.59 69.13,33.59 70.21,34.67 70.21,40.89 69.51,41.59 68.94,41.59 | 68.94,33.59 68.94,33.4 | 68.94,33.4 v68.94,31.88 | 68.94,41.59 68.94,41.78 | 68.94,41.78 v68.94,43.56 | J1.2 68.94,41.59 | 68.94,41.78 68.75,41.59 | 68.94,41.78 69.13,41.59 | 68.94,33.4 68.75,33.59 | 68.94,33.4 69.13,33.59
  Bottom 0.127: J5.1 12.67,10.08 v12.62,10.03 | FG1.10 69.23,31.59 v68.94,31.88 | FG1.2 68.97,43.59 v68.94,43.56 | v50.6,30.35 v50.6,27.3 50.98,26.92 50.98,23.75 52.25,22.48 52.37,22.35 52.4,22.32 J3.15 | v19.23,13.72 19.23,18.8 20.62,20.19 20.62,22.22 J3.66
SDA  (via drill 0.25 pad 0.51)
  Top 0.127: J4.2 16.67,13.48 16.43,13.72 v15.67,13.72 | v53.14,27.81 22.4,27.81 19.38,24.79 J3.68 | J1.3 68.77,40.59 68.94,40.77 v68.94,40.89 69.83,40.01 69.83,35.31 v68.94,34.42 68.77,34.59 J1.9 64.74,34.59 64.44,34.29 64.44,33.27 62.03,30.86 v53.14,30.86
  Bottom 0.127: J5.2 14.67,13.35 15.04,13.72 v15.67,13.72 15.67,17.14 16.69,18.16 16.69,18.54 17.96,19.81 17.96,20.45 19.35,21.84 19.35,24.12 J3.68 | FG1.9 69.25,33.09 68.94,33.4 v68.94,34.42 | FG1.3 69.25,42.09 68.94,41.78 v68.94,40.89 | v53.14,30.86 v53.14,27.81 53.77,27.18 53.77,23.75 54.79,22.73 54.79,21.84 53.67,20.73 J3.13
VCC  (via drill 0.25 pad 0.51)
  Top 0.406: D6.+ 1.82,29.96 2.33,30.48 12.75,30.48 15.29,33.02 15.29,45.97 15.29,46.1
  Top 0.508: v15.04,46.23 15.04,46.1 15.16,45.97
  Top 1.016: v24.69,46.61 v24.69,45.97 24.69,45.85 23.42,44.58 17.32,44.58 15.92,45.97 15.29,45.97 15.16,45.97
  Bottom 0.305: U6.7 16.44,46.61 16.3,46.48 | 16.3,46.48 16.05,46.48 | 16.05,46.48 15.8,46.48 | U6.8 15.94,46.6 16.05,46.48 | 16.3,46.48 16.3,45.97
  Bottom 1.016: D5.+ v24.69,45.97
  other vias: 15.67,46.23
  pour Bottom (isolate 0.254, no thermals): 14.78,47.73 14.78,48.35 13.98,49.15 12.24,49.15 12.11,49.02 12.11,47.88 12.24,47.75 12.65,47.75 14.02,46.38 14.02,45.72 14.15,45.59 14.91,45.59 15.16,45.34 15.16,44.2 15.42,43.94 16.43,43.94 16.56,44.07 16.56,45.97 16.05,46.48 16.05,47.24 15.92,47.37 15.14,47.37
VOUT  (via drill 0.25 pad 0.51)
  Top 0.508: J1.4 68.91,39.59 v68.94,39.62 | v68.94,35.56 68.91,35.59 J1.8 64.6,35.59 v64.56,35.56
  Top 0.61: J1.4 64.91,39.59 | 64.91,39.59 64.53,39.59 v64.31,39.37 | 64.91,39.59 64.56,39.24
  Top 1.016: v64.31,38.61 v64.31,39.37 64.31,39.62 | v26.46,51.05 60.76,51.05 v62.91,48.9
  Bottom 0.406: R4.2 D4.-
  Bottom 0.508: v68.94,39.62 68.94,39.88 69.65,40.59 FG1.4 | FG1.8 69.78,34.59 68.94,35.43 v68.94,35.56
  Bottom 1.016: D4.- D5.- v26.46,51.05 v27.23,51.05 | v64.56,35.56 64.31,35.81 v64.31,38.61 v64.31,39.37 64.31,40.01 62.91,41.4 C5.2 C6.2 v62.91,48.9 v62.41,49.4

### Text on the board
tNames: GND | 3V3 | P8 | P0 | USB | Micro | PWR | P12 | GND | 3V3 | SDA | SCL | GND | 3V3 | P14 | P0 | GND | 3V3 | P15 | P1 | GND | 3V3 | P16 | P2 | P1 | P13 | P2 | I2C | P0/P14 | P1/P15 | P2/P16
bNames: v1.2 | SCL | SDA | 3V3 | GND | P12 | NC | 3V3 | GND | P13 | NC | 3V3 | GND | P8 | NC | 3V3 | GND | I2C | P12 | P13 | P8
tTest: BBC micro:bit

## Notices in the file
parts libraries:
moudle-new: This work is licensed under the Creative Commons Attribution 4.0 International License.
To view a copy of this license,visit:
http://creativecommons.org/licenses/by-sa/4.0
moudle-new: CC-BY-SA
